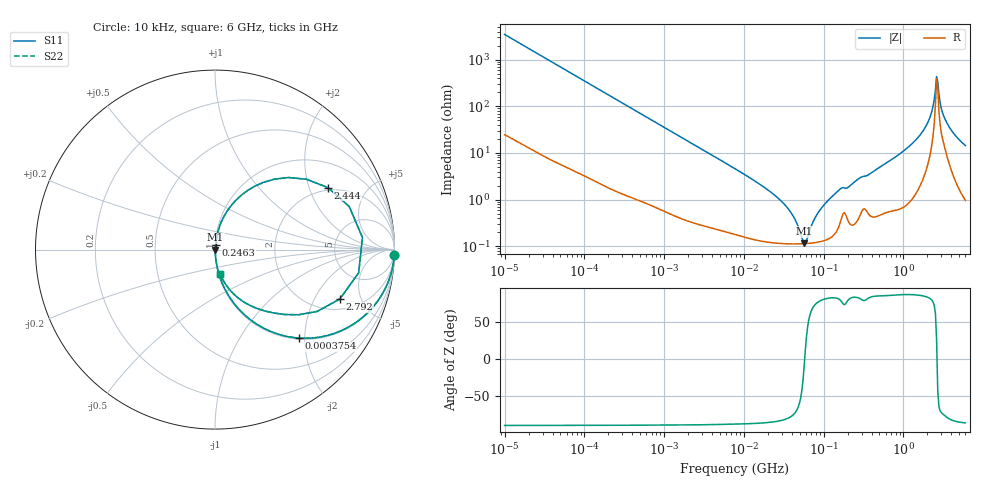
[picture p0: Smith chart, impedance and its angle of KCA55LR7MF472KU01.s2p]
!Murata Part Number: KCA55LR7MF472KU01
!These Parameters are Measured in Series Mode Connection
!Data Generated on Jan 08, 2026
!  o--ll--o
!Port1  Port2
!  o------o
!Operation Temp=25[degC], DC Bias Voltage=0[V]
!Freq. Start=10[kHz] Stop=6[GHz] 401[Steps]
# Hz S RI R 50
!Freq.(Hz) S11(Real) S11(Imag) S21(Real) S21(Imag) S12(Real) S12(Imag) S22(Real) S22(Imag)
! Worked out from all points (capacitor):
!   401 points, 10 kHz to 6 GHz, reference 50 ohm
!   read as one part in series: C = 4.6 nF near 10.69 kHz
!   lowest |Z| = 116 mohm at 56.99 MHz (marker M1)
!   series resonance near 57.96 MHz, so ESL is about 1.6 nH
!   S11 on the Smith chart (normalised r, x): 10 kHz: 1, -69; 375.4 kHz: 1.02, -1.88; 246.3 MHz: 1.01, +0.05; 2.444 GHz: 1.89, +2.69; 2.792 GHz: 2.61, -3.27; 6 GHz: 1.02, -0.29
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10000  0.999 -0.0289  0.00104 0.0289  0.00104 0.0289  0.999 -0.0289
92862  0.932 -0.2471  0.068 0.2471  0.068 0.2471  0.932 -0.2471
180613  0.788 -0.4038  0.212 0.4038  0.212 0.4038  0.788 -0.4038
375445  0.4684 -0.493  0.5316 0.493  0.5316 0.493  0.4684 -0.493
862344  0.1484 -0.3479  0.8516 0.3479  0.8516 0.3479  0.1484 -0.3479
7745967  0.00388 -0.0457  0.9961 0.0457  0.9961 0.0457  0.00388 -0.0457
3.13171e7  0.00121 -0.00828  0.9988 0.00828  0.9988 0.00828  0.00121 -0.00828
4.224642e7  0.00114 -0.00407  0.9989 0.00407  0.9989 0.00407  0.00114 -0.00407
5.698996e7  0.00114 -0.000212  0.9989 0.000212  0.9989 0.000212  0.00114 -0.000212
6.091007e7  0.00115 0.000634  0.9989 -0.000634  0.9989 -0.000634  0.00115 0.000634
7.193098e7  0.00118 0.00278  0.9988 -0.00278  0.9988 -0.00278  0.00118 0.00278
1.184668e8  0.00158 0.0101  0.9984 -0.0101  0.9984 -0.0101  0.00158 0.0101
2.462606e8  0.00356 0.0239  0.9964 -0.0239  0.9964 -0.0239  0.00356 0.0239
6.67969e8  0.00987 0.0658  0.9901 -0.0658  0.9901 -0.0658  0.00987 0.0658
1.752557e9  0.0979 0.2545  0.9021 -0.2545  0.9021 -0.2545  0.0979 0.2545
2.212024e9  0.3299 0.3923  0.6701 -0.3923  0.6701 -0.3923  0.3299 0.3923
2.44414e9  0.6288 0.3456  0.3712 -0.3456  0.3712 -0.3456  0.6288 0.3456
2.612262e9  0.8215 0.0672  0.1785 -0.0672  0.1785 -0.0672  0.8215 0.0672
2.791949e9  0.6954 -0.2754  0.3046 0.2754  0.3046 0.2754  0.6954 -0.2754
3.084918e9  0.3875 -0.3615  0.6125 0.3615  0.6125 0.3615  0.3875 -0.3615
3.643096e9  0.174 -0.2999  0.826 0.2999  0.826 0.2999  0.174 -0.2999
6e9  0.0292 -0.1384  0.9708 0.1384  0.9708 0.1384  0.0292 -0.1384
